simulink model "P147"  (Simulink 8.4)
settings: Solver=ode45  StartTime=0.0  StopTime=10e-3  RelTol=1e-3
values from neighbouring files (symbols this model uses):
  E = (0:1/2:5)'    [IEDummyEx.m]    (also in Test01.m = sum((ObDat-y).^2); TestRtd02.m = sum((ObDat-y).^2))
  R = 1e3    (= 1000)    [IEDummyEx.m]
undefined symbols (not defined in the file or in its folder): C, L

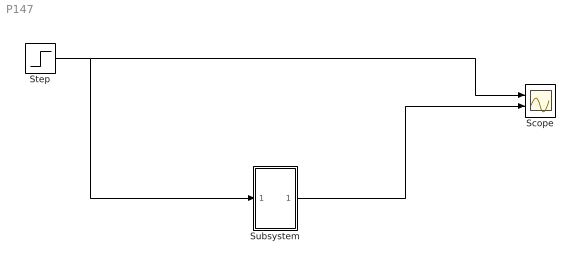
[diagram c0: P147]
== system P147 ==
  Scope : Scope  NumInputPorts=2
  Step : Step  Time=0.001  After=E  SampleTime=0.00001
  Subsystem : Subsystem
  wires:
  Step/1 -> Subsystem/1(In1), Scope/1
  Subsystem/1(Out1) -> Scope/2

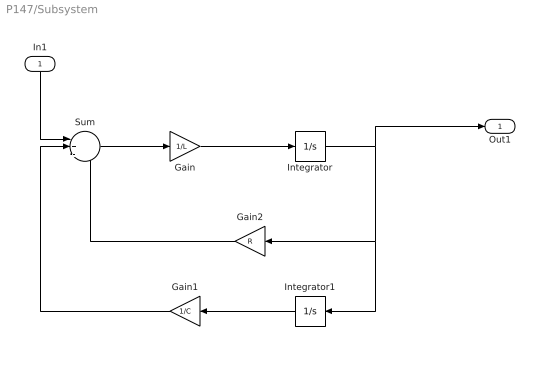
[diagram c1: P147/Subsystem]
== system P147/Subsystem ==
  In1 : Inport
  Gain : Gain  Gain=1/L
  Gain1 : Gain  Gain=1/C
  Gain2 : Gain  Gain=R
  Integrator : Integrator
  Integrator1 : Integrator
  Sum : Sum  Inputs=|+--
  Out1 : Outport
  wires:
  Integrator/1 -> Out1/1, Integrator1/1, Gain2/1
  Gain/1 -> Integrator/1
  Sum/1 -> Gain/1
  Integrator1/1 -> Gain1/1
  Gain1/1 -> Sum/2
  Gain2/1 -> Sum/3
  In1/1 -> Sum/1
